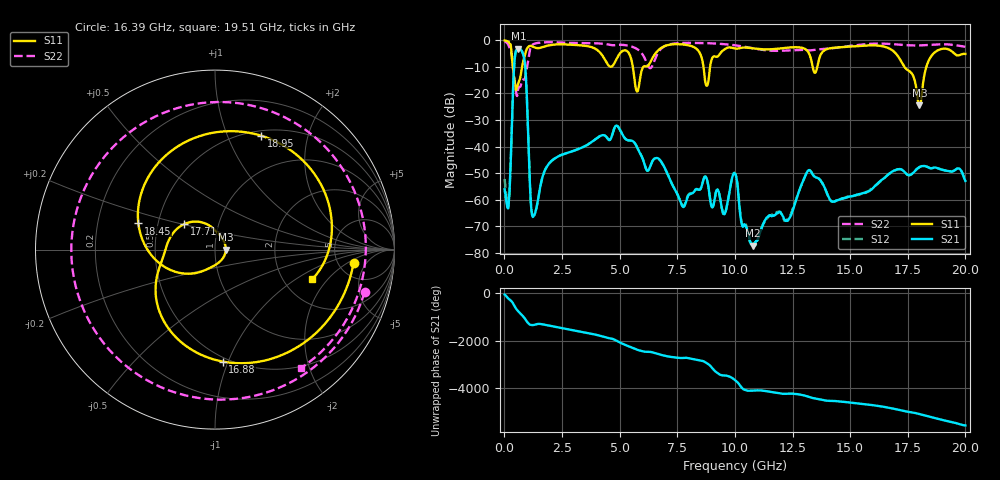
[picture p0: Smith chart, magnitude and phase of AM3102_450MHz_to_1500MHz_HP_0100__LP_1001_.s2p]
!Agilent Technologies,E8364B,MY43040894,A.07.50.67
!Agilent E8364B: A.07.50.67
!Date: Thursday, January 11, 2018 05:37:26
!Correction: S11(Full 2 Port(1,2))
!S21(Full 2 Port(1,2))
!S12(Full 2 Port(1,2))
!S22(Full 2 Port(1,2))
!S2P File: Measurements: S11, S21, S12, S22:
# Hz S  dB  R 50
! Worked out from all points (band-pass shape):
!   1601 points, 10 MHz to 20 GHz, reference 50 ohm
!   highest |S21| = -3.15 dB at 609.7 MHz (marker M1); lowest = -77.3 dB at 10.79 GHz (marker M2)
!   |S21| within 3 dB of the highest: 457 MHz to 839.8 MHz (382.8 MHz wide, 59 % of centre)
!   lowest |S11| = -24.4 dB at 18 GHz (marker M3), VSWR 1.13, Z = 56.4 + j0.0404 ohm
!   |S11| at or under -10 dB: 364.8 MHz to 764 MHz (399.2 MHz wide, 70.7 % of centre); 5.572 GHz to 6.028 GHz (455.7 MHz wide, 7.86 % of centre); 17.36 GHz to 18.31 GHz (950.6 MHz wide, 5.33 % of centre)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
!   |S22| runs from -21.0 to -0.5 dB; largest |S21 - S12| = 0.0016
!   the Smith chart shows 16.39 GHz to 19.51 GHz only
!   S11 on the Smith chart (normalised r, x): 16.39 GHz: 6.97, -2.54; 16.88 GHz: 0.47, -0.96; 17.71 GHz: 0.68, +0.20; 18.45 GHz: 0.39, +0.14; 18.95 GHz: 0.56, +1.33; 19.51 GHz: 2.88, -1.39
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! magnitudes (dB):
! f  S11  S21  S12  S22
! 10 MHz  -0.1  -56.1  -52.2  -0.5
! 184.9 MHz  -0.6  -61.8  -61.3  -2.0
! 434.8 MHz  -14.9  -8.3  -8.3  -14.6
! 609.7 MHz  -16.0  -3.2  -3.2  -18.0
! 884.6 MHz  -5.7  -8.4  -8.4  -14.6
! 1.259 GHz  -2.5  -66.3  -65.9  -1.4
! 3.346 GHz  -1.9  -40.5  -40.5  -1.1
! 5.757 GHz  -19.3  -40.3  -40.3  -3.3
! 6.682 GHz  -3.7  -44.5  -44.6  -4.5
! 7.756 GHz  -1.6  -62.7  -62.6  -1.0
! 10.01 GHz  -3.1  -50.1  -50.0  -1.9
! 10.79 GHz  -3.0  -77.3  -77.3  -3.0
! 13.34 GHz  -8.6  -49.9  -50.0  -3.7
! 16.39 GHz  -2.2  -52.5  -52.5  -1.2
! 16.68 GHz  -3.0  -50.3  -50.4  -1.3
! 16.88 GHz  -4.1  -49.2  -49.3  -1.5
! 17.71 GHz  -13.0  -50.1  -50.0  -1.9
! 18 GHz  -24.4  -47.8  -47.8  -1.9
! 18.45 GHz  -6.9  -48.1  -48.1  -1.7
! 18.95 GHz  -3.3  -48.6  -48.6  -1.5
! 19.51 GHz  -4.9  -49.1  -49.0  -1.8
! 20 GHz  -5.1  -52.9  -52.8  -2.4
